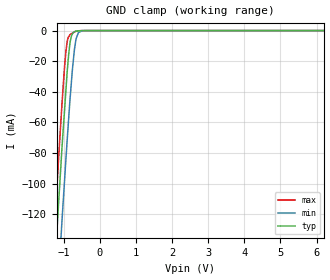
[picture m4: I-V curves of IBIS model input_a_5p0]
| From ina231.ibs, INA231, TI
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|   input_a_5p0 Model
[Model]   input_a_5p0
Model_type   Input
Vinl = 0.4
Vinh = 1.4
|   typ   min   max
|   (nom PVT)   (fast PVT)   (slow PVT)
|C_comp from frequency sweep method (F=100KHz)
|Average
|C_comp   1.113e-12   8.846e-13   1.380e-12
|C_comp from LC tank measurement(L=1nH)
|Average
|Resonant Frequency(Hz)   9.150e+09   9.580e+09   8.540e+09
C_comp   3.029e-13   2.763e-13   3.477e-13
| Where nom  PVT is Nominal Process, 5V, 27C
|   Fast PVT is Strong Process,  5.5V, -40C
|   Slow PVT is Weak Process,   4.5V, 125C
[Voltage Range]   5   4.5   5.5
|Ambient Temperature   25   150   -65
|Junction Temperature
[Temperature Range]   27   125   -40
[Power Clamp Reference]   5   4.5   5.5
[GND Clamp Reference]   0   0   0
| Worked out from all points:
|   GND clamp passes 1 mA (typ) near -0.72 V on its own axis
[GND Clamp]
|   Voltage   I(typ)   I(min)   I(max)
-5V       -1.739A    -1.766A    -1.726A
-1.368V   -203mA     -249.8mA   -174.9mA
-1.192V   -132.6mA   -180mA     -103.9mA
-1.122V   -104.7mA   -152.7mA   -75.46mA
-1.045V   -75.21mA   -123mA     -46.51mA
-940.5mV  -39.15mA   -84.2mA    -13.74mA
-902mV    -26.01mA   -70.49mA   -6.83mA
-820mV    -7.061mA   -43.07mA   -2.518mA
-670mV    -393.1uA   -6.949mA   -526.6uA
-589.5mV  -216.1uA   -1.251mA   -133uA
-369mV    -1.371uA   -6.535uA   -7.947uA
10V       0A         0A         0A
[POWER Clamp]
|   Voltage   I(typ)   I(min)   I(max)
-5V       0A         0A         0A
-5V       0A         0A         0A
10V       0A         0A         0A
